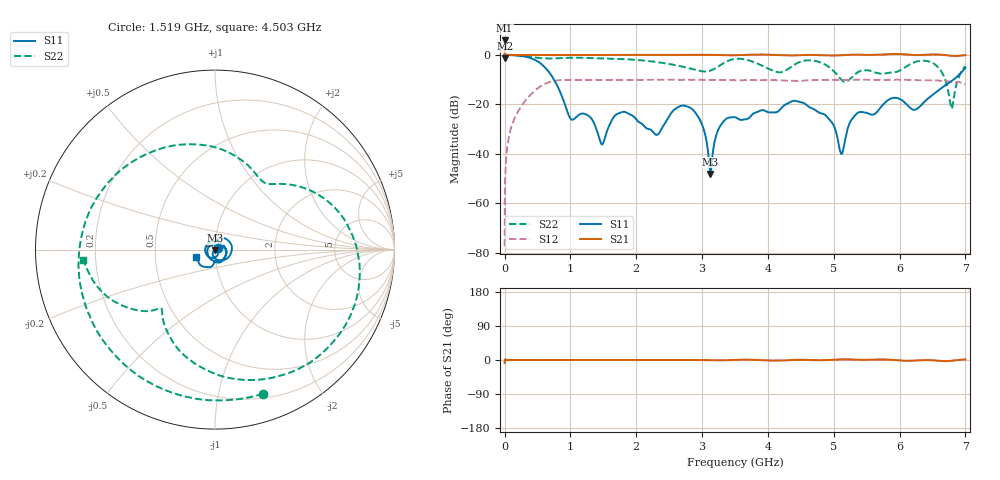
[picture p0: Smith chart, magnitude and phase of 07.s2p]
!Keysight Technologies,N5232A,MY52221221,A.10.65.11
!Date: Wednesday, October 16, 2024 11:54:56
!Correction: S11(Full 2 Port(1,4))
!S41(Full 2 Port(1,4))
!S14(Full 2 Port(1,4))
!S44(Full 2 Port(1,4))
!S2P File: Measurements: S11, S41, S14, S44:
# Hz S  RI  R 50
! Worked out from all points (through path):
!   4001 points, 300 kHz to 7 GHz, reference 50 ohm
!   highest |S21| = 5.85 dB at 300 kHz (marker M1); lowest = -1.3 dB at 2.05 MHz (marker M2)
!   lowest |S11| = -48.1 dB at 3.127 GHz (marker M3), VSWR 1.01, Z = 50 - j0.392 ohm
!   |S11| at or under -10 dB: 750.9 MHz to 6.819 GHz (6.068 GHz wide, 160 % of centre)
!   |S22| runs from -21.8 to 0.0 dB; largest |S21 - S12| = 2
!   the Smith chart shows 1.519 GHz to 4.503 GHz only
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300000  -0.9929 -0.0136  1.944 -0.2639  4.59e-05 0.000129  -0.989 -0.0217
2049925  -0.969 0.1506  0.8578 -0.0121  0.000136 0.000698  -0.9771 0.0976
7.554678e7  -0.8001 0.5932  0.9938 -0.00278  0.0128 0.0223  -0.9648 0.2445
2.032913e8  0.1526 0.9589  1.001 -0.00113  0.0708 0.0114  -0.7664 0.5969
3.415354e8  0.8921 0.1672  0.9997 0.0012  0.0874 -0.0978  -0.4306 0.8295
4.867792e8  0.281 -0.7087  0.9994 -0.00117  -0.0804 -0.1876  -0.0506 0.8794
6.320229e8  -0.4586 -0.2606  0.9981 0.00089  -0.2681 0.01  0.2699 0.8055
1.1675e9  0.0299 0.0578  0.9986 0.00189  0.1666 -0.2643  0.8469 -0.2168
1.478987e9  0.0155 0.000784  0.9994 0.00242  -0.312 0.0119  0.3579 -0.7709
1.687228e9  0.061 -0.00248  0.9994 0.00285  -0.0327 0.3099  -0.1274 -0.8268
2.3347e9  -0.000246 0.0251  1.003 -0.000137  -0.2872 -0.1292  -0.6373 0.3195
2.819429e9  0.074 -0.0438  1.004 -0.000359  0.3014 0.0903  0.1152 0.5199
3.127416e9  0.000492 -0.00392  1.005 -0.00875  -0.066 -0.3066  0.3145 0.3653
3.50015e9  -0.0546 0.00694  0.9852 0.0049  -0.1262 0.281  0.7944 -0.2458
3.792387e9  0.064 -0.0195  1.015 0.00716  0.3113 0.0128  0.0619 -0.7123
4.257868e9  -0.021 -0.0956  0.977 -0.0185  -0.301 -0.0143  -0.3378 -0.3364
4.66735e9  -0.0821 0.0145  0.999 -0.003  0.2726 0.1424  -0.6188 0.4644
5.118831e9  0.0092 -0.00405  0.9871 0.0268  -0.2647 -0.1689  0.1643 0.2657
5.83455e9  -0.087 0.0899  1.035 0.0199  0.1246 -0.287  0.4095 -0.1463
6.497772e9  0.00799 0.1546  1.023 -0.0129  0.2737 0.1411  -0.6309 -0.288
6.790009e9  0.2862 -0.0708  0.9611 -0.0344  -0.0236 -0.2935  -0.0817 -0.00268
7e9  -0.4427 -0.3187  0.992 0.0257  -0.2499 0.0475  -0.5911 -0.0499
